(* Logix 5000 AddOnInstructionDefinition export HI1734_Faceplate_Standard_AOI; software revision 30.00 *)

ADD_ON_INSTRUCTION HI1734_Faceplate_Standard_AOI   (* revision 1.3, vendor Hardy Process solutions *)
// for standard data from module
VAR_IN_OUT
   Inp_hi1734 : HI:1734_WS:I:0; {required}   // Module Input table
   Out_hi1734 : HI:1734_WS:O:0; {required}   // Module Output table
END_VAR
VAR_OUTPUT
   cal_status : SINT; {access Read Only}   // Calibration status indication
   hardy_1734_ints_st : INT;   // Instrument Status
END_VAR
VAR_INPUT
   fp_dis_md : INT;   // display mode gross/net
   tare_cmd : BOOL;   // Tare cmd trigger
   zero_cmd : BOOL;   // Zero cmd trigger
END_VAR
VAR_OUTPUT
   hardy_1734_net_wt : REAL;   // Net weight
   hardy_1734_gross_wt : REAL;   // Gross weight
END_VAR
VAR_INPUT
   rd_fill : BOOL;   // Read Filter parameter trigger
   pm_2081 : DINT;   // WAVERSAVER
   rd_az : BOOL;   // Read zero parameters trigger
   pm_6301 : DINT;   // Auto Zero Enable
   pm_6302 : REAL;   // Auto Zero tolerance
   pm_6201 : REAL;   // zero'd weight
   pm_2886 : REAL;   // Zero Tolerance
   pm_6183 : REAL;   // Tare Weight
   rd_inst : BOOL;   // Read Instrument setup parameter trigger
   pm_2881 : DINT;   // Units of measure
   pm_2887 : REAL;   // Motion Tolerance
   rd_c2cal : BOOL;   // Read C2 parameter trigger
   pm_4102 : REAL;   // Gravity correction
   rd_tradcal : BOOL;   // Read Traditional cal parameter trigger
   pm_4182 : REAL;   // Span Weight
   cal_low_cmd : BOOL;   // Cal Low cmd trigger
   cal_high_cmd : BOOL;   // Cal High cmd trigger
   c2_cmd : BOOL;   // C2 cal trigger
END_VAR
VAR_OUTPUT
   status1 : INT;   // Instrument status
END_VAR
VAR_INPUT
   save_c2_pm : BOOL;   // Save C2 setup parameters trigger
   pm_4101 : REAL;   // Ref Weight
   save_tradcal_pm : BOOL;   // Save traditional calibration settings trigger
   save_fil_pm : BOOL;   // Save Filter settings trigger
   save_az_pm : BOOL;   // Save zero parameters trigger
   save_ins_pm : BOOL;   // Save Instrument setup settings trigger
   Set_FaceplateAnimation : INT;   // panel selection on faceplate
   pm_2082 : DINT;   // Num Averages
END_VAR
VAR_OUTPUT
   cmd_status : DINT; {access Read Only}   // Command status indication
END_VAR
VAR_INPUT
   reset_waversaver_indicator : BOOL;   // Reset WAVERSAVER selection indication on faceplate
   reset_az_enable_indication : BOOL;   // Reset auto zero selection indication on faceplate
   reset_units_indication : BOOL;   // Reset units selection indication on faceplate
   percent_weight : REAL;   // percentage of scale capacity for trend screen
   pm_2888 : REAL;   // scale capacity used for trend
END_VAR
VAR
   start_delay_rd_filter : BOOL; {access None}   // processs control bit
   delay_rd_filter : TIMER := (PRE := 200); {access None}   // Delay timer to allow time for process to complete
   rd_inst2 : BOOL; {access None}   // processs control bit
   wr_C2_ref_wt_1 : BOOL; {access None}   // processs control bit
   wr_gravity_correction_1 : BOOL; {access None}   // processs control bit
   wr_span_wt_1 : BOOL; {access None}   // processs control bit
   wr_waversaver_1 : BOOL; {access None}   // processs control bit
   wr_number_avgerages_1 : BOOL; {access None}   // processs control bit
   wr_zero_tolerance_1 : BOOL; {access None}   // processs control bit
   wr_tare_weight_1 : BOOL; {access None}   // processs control bit
   wr_motion_tolerance_1 : BOOL; {access None}   // processs control bit
   wr_units_measure_1 : BOOL; {access None}   // processs control bit
   start_delay_rd_zero_1 : BOOL; {access None}   // processs control bit
   delay_rd_zero_1 : TIMER := (PRE := 200); {access None}   // Delay timer to allow time for process to complete
   start_delay_rd_zero_2 : BOOL; {access None}   // processs control bit
   delay_rd_zero_2 : TIMER := (PRE := 200); {access None}   // Delay timer to allow time for process to complete
   start_delay_rd_inst_1 : BOOL; {access None}   // processs control bit
   delay_rd_inst_1 : TIMER := (PRE := 200); {access None}   // Delay timer to allow time for process to complete
   wr_auto_zero_enable_1 : BOOL; {access None}   // processs control bit
   wr_auto_zero_tolerance_1 : BOOL; {access None}   // processs control bit
   start_delay_rd_inst_2 : BOOL; {access None}   // processs control bit
   delay_rd_inst_2 : TIMER := (PRE := 200); {access None}   // Delay timer to allow time for process to complete
   start_delay_rd_C2cal : BOOL; {access None}   // processs control bit
   delay_rd_C2cal : TIMER := (PRE := 200); {access None}   // Delay timer to allow time for process to complete
   start_delay_rd_tradcal : BOOL; {access None}   // processs control bit
   delay_rd_tradcal : TIMER := (PRE := 200); {access None}   // Delay timer to allow time for process to complete
   cmd_no : INT; {access None}   // Cmd number being sent to module
   run_cmd : BOOL; {access None}   // processs control bit
   chec_status_wr_C2_ref : BOOL; {access None}   // triggers status check of write C2 ref
   start_delay_wr_C2_ref : BOOL; {access None}   // processs control bit
   delay_wr_C2_ref : TIMER := (PRE := 200); {access None}   // Delay timer to allow time for process to complete
   check_status_wr_gravity_correction : BOOL; {access None}   // triggers status check of write of parameter
   start_delay_wr_gravity_correction : BOOL; {access None}   // processs control bit
   delay_wr_gravity_correction : TIMER := (PRE := 200); {access None}   // Delay timer to allow time for process to complete
   wr_traditional_ref_wt_1 : BOOL; {access None}   // processs control bit
   check_status_wr_traditional_ref : BOOL; {access None}   // triggers status check of write of parameter
   start_delay_wr_traditional_ref : BOOL; {access None}   // processs control bit
   delay_wr_traditional_ref : TIMER := (PRE := 200); {access None}   // Delay timer to allow time for process to complete
   check_status_wr_span_wt : BOOL; {access None}   // triggers status check of write of parameter
   start_delay_wr_span_wt : BOOL; {access None}   // processs control bit
   delay_wr_span_wt : TIMER := (PRE := 200); {access None}   // Delay timer to allow time for process to complete
   check_status_wr_waversaver : BOOL; {access None}   // triggers status check of write of parameter
   start_delay_wr_waversaver : BOOL; {access None}   // processs control bit
   delay_wr_waversaver : TIMER := (PRE := 200); {access None}   // Delay timer to allow time for process to complete
   check_status_wr_averages : BOOL; {access None}   // triggers status check of write of parameter
   start_delay_wr_averages : BOOL; {access None}   // processs control bit
   delay_wr_averages : TIMER := (PRE := 200); {access None}   // Delay timer to allow time for process to complete
   initial_unit_rd : BOOL; {access None}   // initial read to set up initial display of units.
   check_status_wr_zero_tolerance : BOOL; {access None}   // triggers status check of write of parameter
   start_delay_wr_zero_tolerance : BOOL; {access None}   // processs control bit
   delay_wr_zero_tolerance : TIMER := (PRE := 200); {access None}   // Delay timer to allow time for process to complete
   check_status_wr_tare_weight : BOOL; {access None}   // triggers status check of write of parameter
   start_delay_wr_tare_weight : BOOL; {access None}   // processs control bit
   delay_wr_tare_weight : TIMER := (PRE := 200); {access None}   // Delay timer to allow time for process to complete
   check_status_wr_auto_zero_enable : BOOL; {access None}   // triggers status check of write parameter
   start_delay_wr_auto_zero_enable : BOOL; {access None}   // processs control bit
   delay_wr_auto_zero_enable : TIMER := (PRE := 200); {access None}   // Delay timer to allow time for process to complete
   start_delay_wr_auto_zero_tolerance : BOOL; {access None}   // processs control bit
   check_status_wr_auto_zero_tolerance : BOOL; {access None}   // triggers status check of write of parameter
   delay_wr_auto_zero_tolerance : TIMER := (PRE := 200); {access None}   // Delay timer to allow time for process to complete
   check_status_wr_motion_tolerance : BOOL; {access None}   // triggers status check of write of parameter
   start_delay_wr_motion_toleranc : BOOL; {access None}   // processs control bit
   delay_wr_motion_toleranc : TIMER := (PRE := 200); {access None}   // Delay timer to allow time for process to complete
   check_status_wr_units_measure : BOOL; {access None}   // triggers status check of write of parameter
   start_delay_wr_units_measure : BOOL; {access None}   // processs control bit
   delay_wr_units_measure : TIMER := (PRE := 200); {access None}   // Delay timer to allow time for process to complete
   start_delay_init_units_rd : BOOL; {access None}   // processs control bit
   delay_init_units_rd : TIMER := (PRE := 200); {access None}   // Delay timer to allow time for process to complete
   run_cmd_delay : TIMER := (PRE := 1000); {access None}   // Delay timer to allow time for process to complete
   rd_zero_2 : BOOL; {access None}   // processs control bit
   wr_C2_ref_wt_2 : BOOL; {access None}   // processs control bit
   wr_gravity_correction_2 : BOOL; {access None}   // processs control bit
   wr_traditional_ref_wt_2 : BOOL; {access None}   // processs control bit
   wr_span_wt_2 : BOOL; {access None}   // processs control bit
   wr_waversaver_2 : BOOL; {access None}   // processs control bit
   wr_number_avgerages_2 : BOOL; {access None}   // processs control bit
   wr_auto_zero_enable_2 : BOOL; {access None}   // processs control bit
   wr_auto_zero_tolerance_2 : BOOL; {access None}   // processs control bit
   wr_zero_tolerance_2 : BOOL; {access None}   // processs control bit
   wr_units_measure_2 : BOOL; {access None}   // processs control bit
   wr_motion_tolerance_2 : BOOL; {access None}   // processs control bit
   wr_tare_weight_2 : BOOL; {access None}   // processs control bit
   ons_1 : BOOL; {access None}   // processs control bit
   ons_2 : BOOL; {access None}   // processs control bit
   ons_3 : BOOL; {access None}   // processs control bit
   ons_4 : BOOL; {access None}   // processs control bit
   ons_5 : BOOL; {access None}   // processs control bit
   ons_6 : BOOL; {access None}   // processs control bit
   ons_7 : BOOL; {access None}   // processs control bit
   ons_8 : BOOL; {access None}   // processs control bit
   ons_9 : BOOL; {access None}   // processs control bit
   ons_10 : BOOL; {access None}   // processs control bit
   ons_11 : BOOL; {access None}   // processs control bit
   ons_12 : BOOL; {access None}   // processs control bit
   ons_13 : BOOL; {access None}   // processs control bit
   ons_14 : BOOL; {access None}   // processs control bit
   ons_15 : BOOL; {access None}   // processs control bit
   delay_reset_waversaer_ind : TIMER := (PRE := 200); {access None}   // Delay timer to allow time for process to complete
   delay_reset_az_enable_indication : TIMER := (PRE := 200); {access None}   // Delay timer to allow time for process to complete
   delay_reset_units_indication : TIMER := (PRE := 200); {access None}   // Delay timer to allow time for process to complete
END_VAR

ROUTINE Logic   (* ladder *)
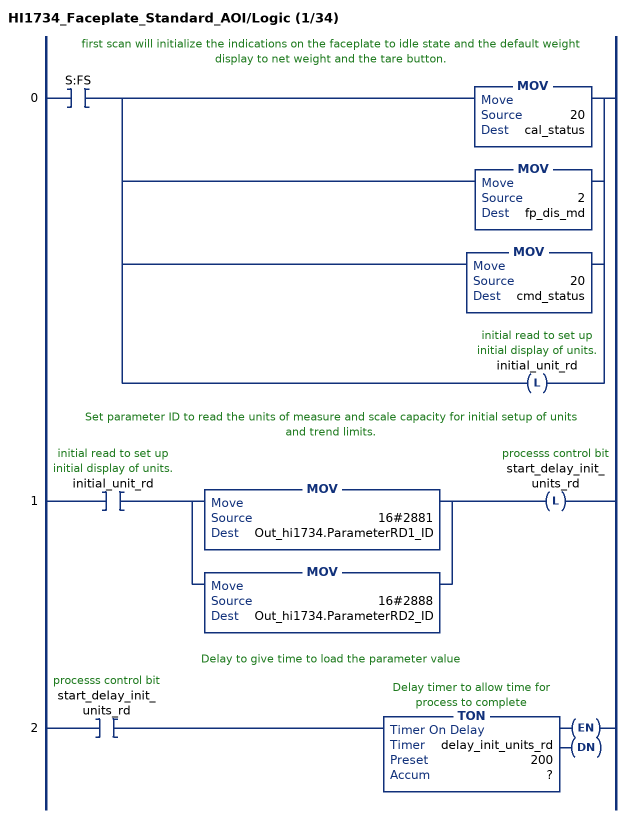
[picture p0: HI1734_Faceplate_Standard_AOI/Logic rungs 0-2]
   // first scan will initialize the indications on the faceplate to idle state and the default weight display to net weight and the tare button.
   0: XIC(S:FS)[MOV(20,cal_status) ,[MOV(2,fp_dis_md) ,MOV(20,cmd_status) ,OTL(initial_unit_rd) ] ];
   // Set parameter ID to read the units of measure and scale capacity for initial setup of units and trend limits.
   1: XIC(initial_unit_rd)[MOV(16#2881,Out_hi1734.ParameterRD1_ID) ,MOV(16#2888,Out_hi1734.ParameterRD2_ID) ]OTL(start_delay_init_units_rd);
   // Delay to give time to load the parameter value
   2: XIC(start_delay_init_units_rd)TON(delay_init_units_rd,?,?);
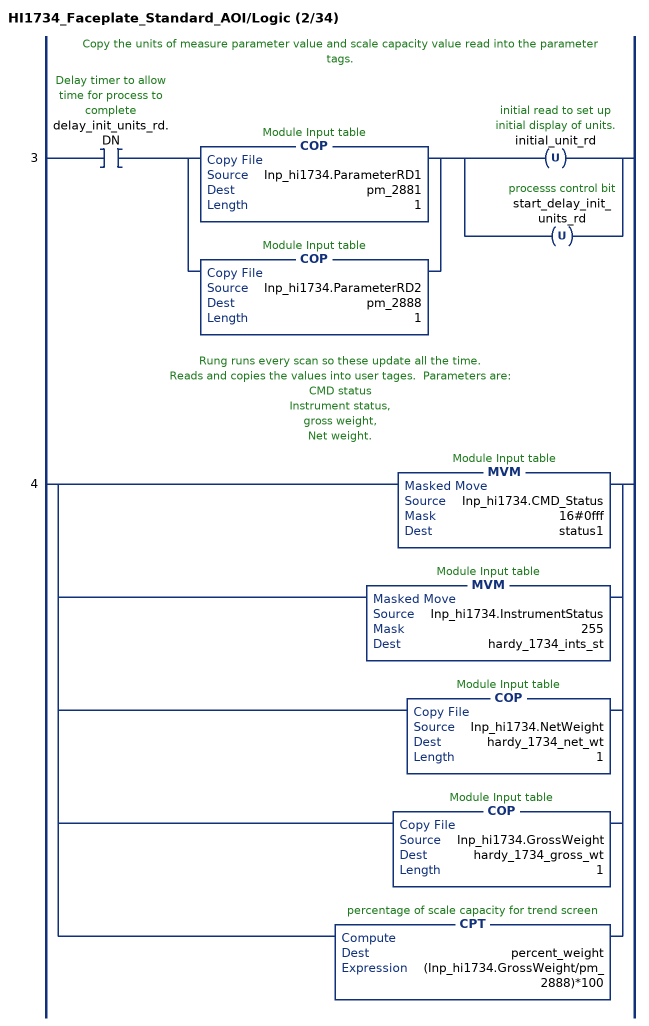
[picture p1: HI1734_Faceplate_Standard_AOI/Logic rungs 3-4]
   // Copy the units of measure parameter value and scale capacity value read into the parameter tags.
   3: XIC(delay_init_units_rd.DN)[COP(Inp_hi1734.ParameterRD1,pm_2881,1) ,COP(Inp_hi1734.ParameterRD2,pm_2888,1) ][OTU(initial_unit_rd) ,OTU(start_delay_init_units_rd) ];
   // Rung runs every scan so these update all the time.
   // Reads and copies the values into user tages.  Parameters are:
   // CMD status
   // Instrument status,
   // gross weight,
   // Net weight.
   4: [MVM(Inp_hi1734.CMD_Status,16#0fff,status1) ,MVM(Inp_hi1734.InstrumentStatus,255,hardy_1734_ints_st) ,COP(Inp_hi1734.NetWeight,hardy_1734_net_wt,1) ,COP(Inp_hi1734.GrossWeight,hardy_1734_gross_wt,1) ,CPT(percent_weight,(Inp_hi1734.GrossWeight/pm_2888)*100) ];
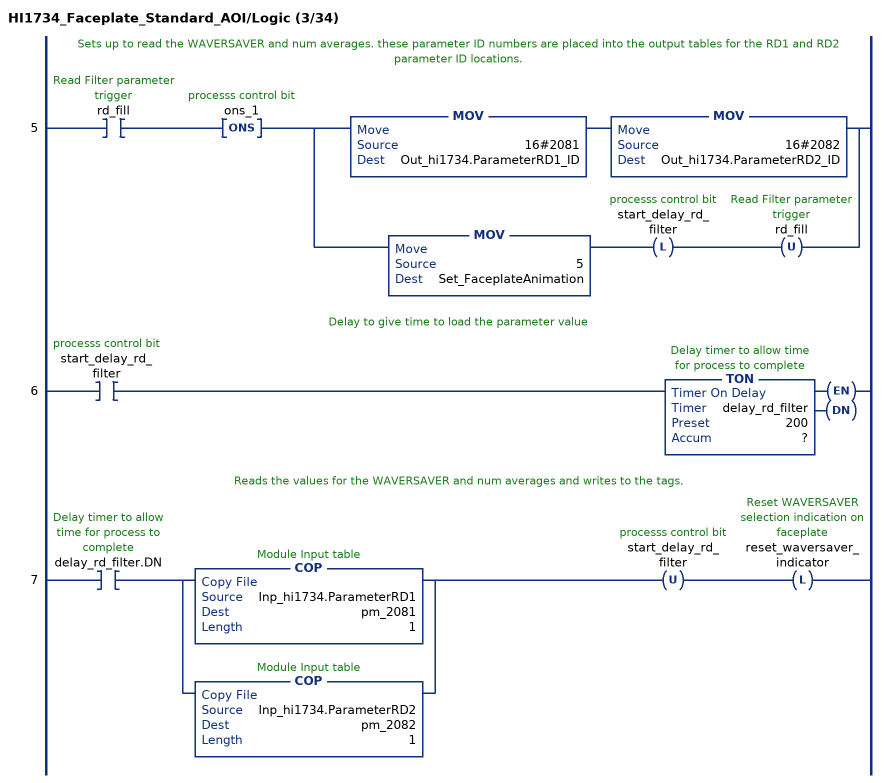
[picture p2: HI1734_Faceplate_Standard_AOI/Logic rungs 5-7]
   // Sets up to read the WAVERSAVER and num averages. these parameter ID numbers are placed into the output tables for the RD1 and RD2 parameter ID locations.
   5: XIC(rd_fill)ONS(ons_1)[MOV(16#2081,Out_hi1734.ParameterRD1_ID) MOV(16#2082,Out_hi1734.ParameterRD2_ID) ,MOV(5,Set_FaceplateAnimation) OTL(start_delay_rd_filter) OTU(rd_fill) ];
   // Delay to give time to load the parameter value
   6: XIC(start_delay_rd_filter)TON(delay_rd_filter,?,?);
   // Reads the values for the WAVERSAVER and num averages and writes to the tags.
   7: XIC(delay_rd_filter.DN)[COP(Inp_hi1734.ParameterRD1,pm_2081,1) ,COP(Inp_hi1734.ParameterRD2,pm_2082,1) ]OTU(start_delay_rd_filter)OTL(reset_waversaver_indicator);
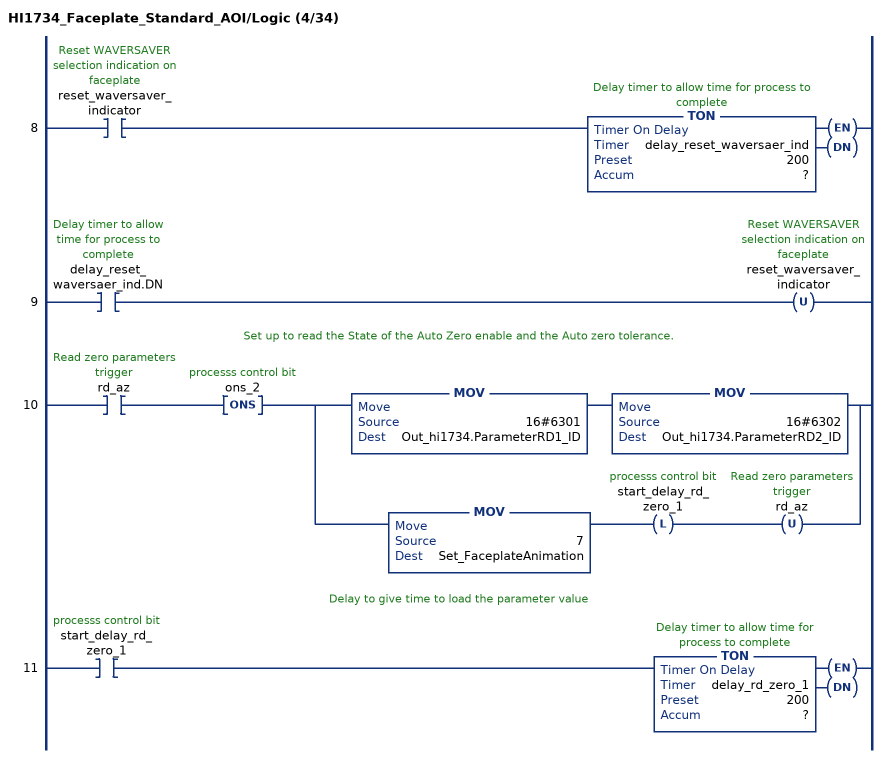
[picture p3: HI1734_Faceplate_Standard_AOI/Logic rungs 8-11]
   8: XIC(reset_waversaver_indicator)TON(delay_reset_waversaer_ind,?,?);
   9: XIC(delay_reset_waversaer_ind.DN)OTU(reset_waversaver_indicator);
   // Set up to read the State of the Auto Zero enable and the Auto zero tolerance.
   10: XIC(rd_az)ONS(ons_2)[MOV(16#6301,Out_hi1734.ParameterRD1_ID) MOV(16#6302,Out_hi1734.ParameterRD2_ID) ,MOV(7,Set_FaceplateAnimation) OTL(start_delay_rd_zero_1) OTU(rd_az) ];
   // Delay to give time to load the parameter value
   11: XIC(start_delay_rd_zero_1)TON(delay_rd_zero_1,?,?);
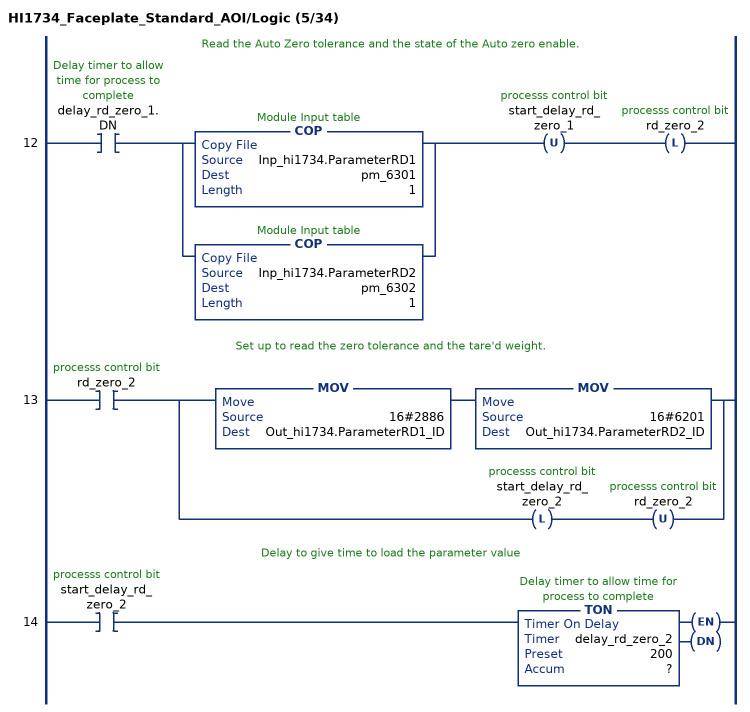
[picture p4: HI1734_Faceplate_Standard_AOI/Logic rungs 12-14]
   // Read the Auto Zero tolerance and the state of the Auto zero enable.
   12: XIC(delay_rd_zero_1.DN)[COP(Inp_hi1734.ParameterRD1,pm_6301,1) ,COP(Inp_hi1734.ParameterRD2,pm_6302,1) ]OTU(start_delay_rd_zero_1)OTL(rd_zero_2);
   // Set up to read the zero tolerance and the tare'd weight.
   13: XIC(rd_zero_2)[MOV(16#2886,Out_hi1734.ParameterRD1_ID) MOV(16#6201,Out_hi1734.ParameterRD2_ID) ,OTL(start_delay_rd_zero_2) OTU(rd_zero_2) ];
   // Delay to give time to load the parameter value
   14: XIC(start_delay_rd_zero_2)TON(delay_rd_zero_2,?,?);
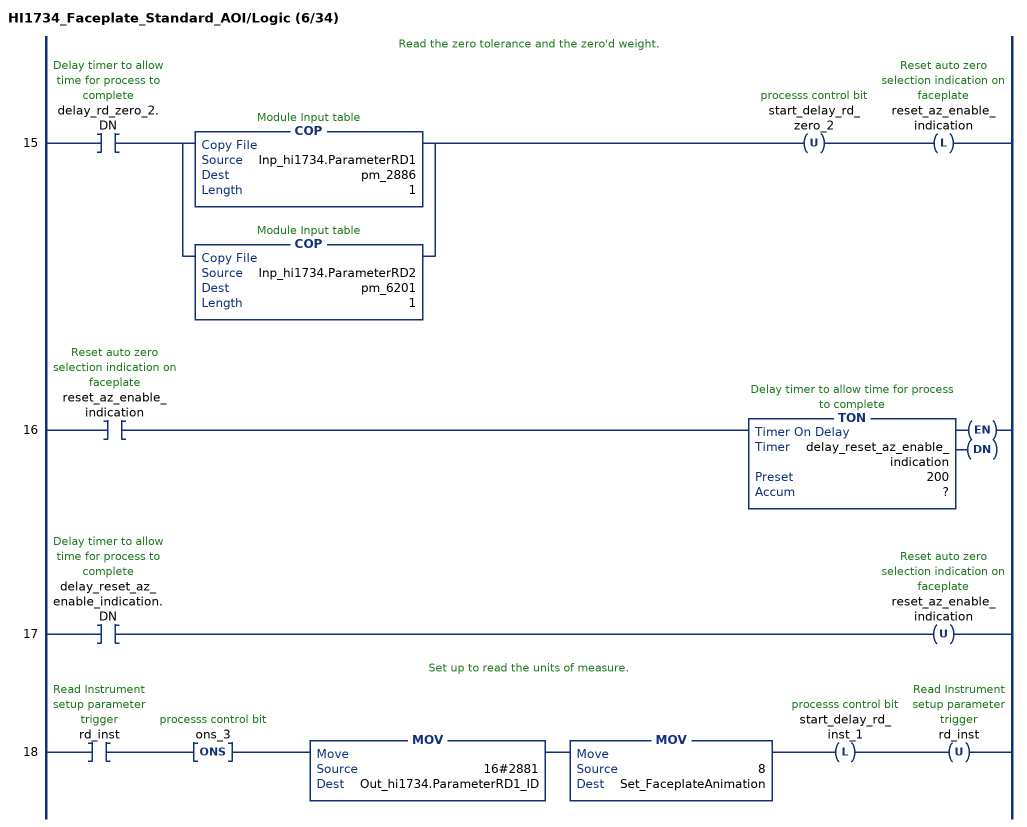
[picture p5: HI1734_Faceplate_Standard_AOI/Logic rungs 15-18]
   // Read the zero tolerance and the zero'd weight.
   15: XIC(delay_rd_zero_2.DN)[COP(Inp_hi1734.ParameterRD1,pm_2886,1) ,COP(Inp_hi1734.ParameterRD2,pm_6201,1) ]OTU(start_delay_rd_zero_2)OTL(reset_az_enable_indication);
   16: XIC(reset_az_enable_indication)TON(delay_reset_az_enable_indication,?,?);
   17: XIC(delay_reset_az_enable_indication.DN)OTU(reset_az_enable_indication);
   // Set up to read the units of measure.
   18: XIC(rd_inst)ONS(ons_3)MOV(16#2881,Out_hi1734.ParameterRD1_ID)MOV(8,Set_FaceplateAnimation)OTL(start_delay_rd_inst_1)OTU(rd_inst);
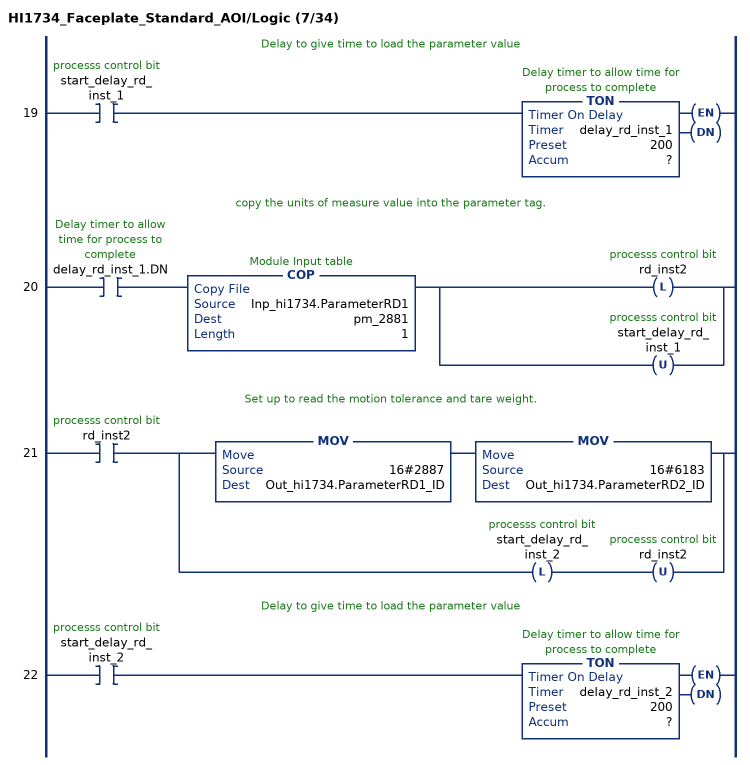
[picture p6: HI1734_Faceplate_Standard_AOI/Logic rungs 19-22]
   // Delay to give time to load the parameter value
   19: XIC(start_delay_rd_inst_1)TON(delay_rd_inst_1,?,?);
   // copy the units of measure value into the parameter tag.
   20: XIC(delay_rd_inst_1.DN)COP(Inp_hi1734.ParameterRD1,pm_2881,1)[OTL(rd_inst2) ,OTU(start_delay_rd_inst_1) ];
   // Set up to read the motion tolerance and tare weight.
   21: XIC(rd_inst2)[MOV(16#2887,Out_hi1734.ParameterRD1_ID) MOV(16#6183,Out_hi1734.ParameterRD2_ID) ,OTL(start_delay_rd_inst_2) OTU(rd_inst2) ];
   // Delay to give time to load the parameter value
   22: XIC(start_delay_rd_inst_2)TON(delay_rd_inst_2,?,?);
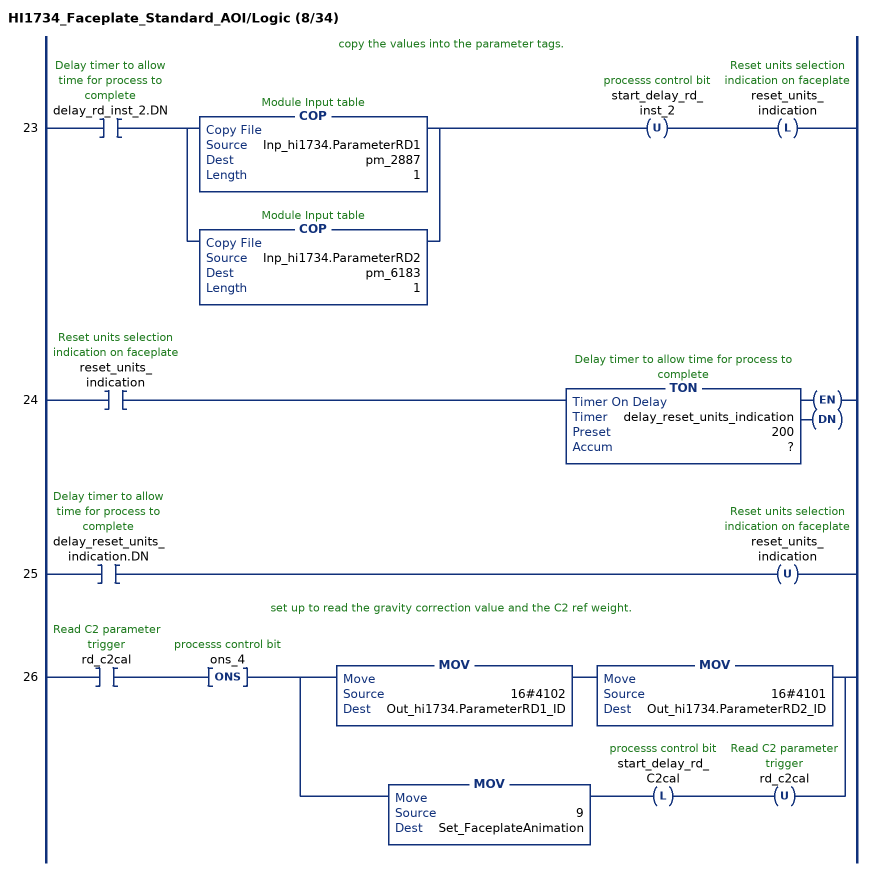
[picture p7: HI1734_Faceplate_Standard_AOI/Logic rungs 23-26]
   // copy the values into the parameter tags.
   23: XIC(delay_rd_inst_2.DN)[COP(Inp_hi1734.ParameterRD1,pm_2887,1) ,COP(Inp_hi1734.ParameterRD2,pm_6183,1) ]OTU(start_delay_rd_inst_2)OTL(reset_units_indication);
   24: XIC(reset_units_indication)TON(delay_reset_units_indication,?,?);
   25: XIC(delay_reset_units_indication.DN)OTU(reset_units_indication);
   // set up to read the gravity correction value and the C2 ref weight.
   26: XIC(rd_c2cal)ONS(ons_4)[MOV(16#4102,Out_hi1734.ParameterRD1_ID) MOV(16#4101,Out_hi1734.ParameterRD2_ID) ,MOV(9,Set_FaceplateAnimation) OTL(start_delay_rd_C2cal) OTU(rd_c2cal) ];
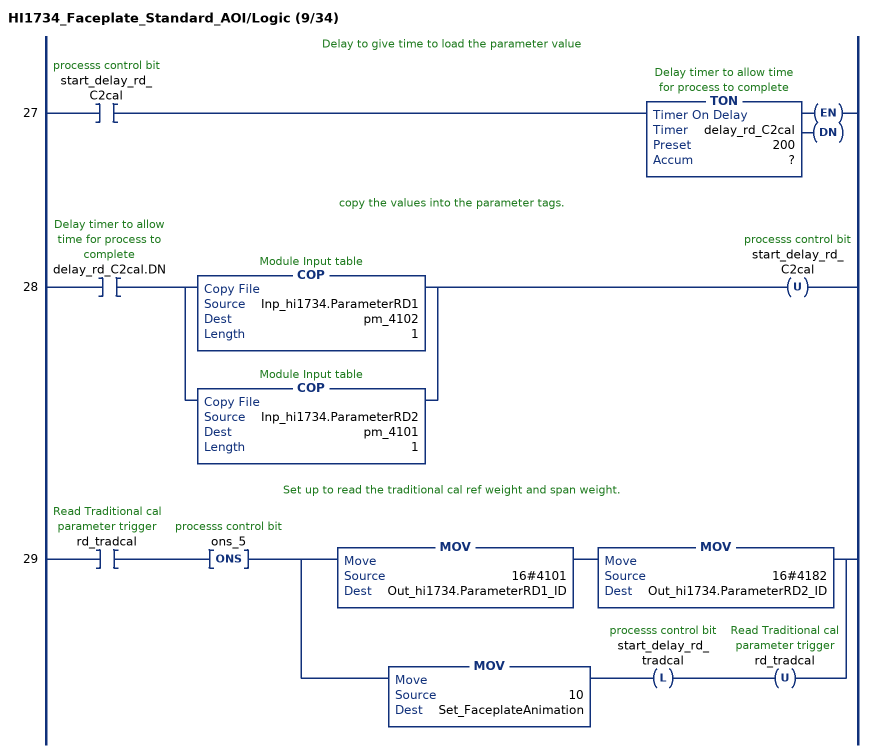
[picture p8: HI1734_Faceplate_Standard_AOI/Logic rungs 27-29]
   // Delay to give time to load the parameter value
   27: XIC(start_delay_rd_C2cal)TON(delay_rd_C2cal,?,?);
   // copy the values into the parameter tags.
   28: XIC(delay_rd_C2cal.DN)[COP(Inp_hi1734.ParameterRD1,pm_4102,1) ,COP(Inp_hi1734.ParameterRD2,pm_4101,1) ]OTU(start_delay_rd_C2cal);
   // Set up to read the traditional cal ref weight and span weight.
   29: XIC(rd_tradcal)ONS(ons_5)[MOV(16#4101,Out_hi1734.ParameterRD1_ID) MOV(16#4182,Out_hi1734.ParameterRD2_ID) ,MOV(10,Set_FaceplateAnimation) OTL(start_delay_rd_tradcal) OTU(rd_tradcal) ];
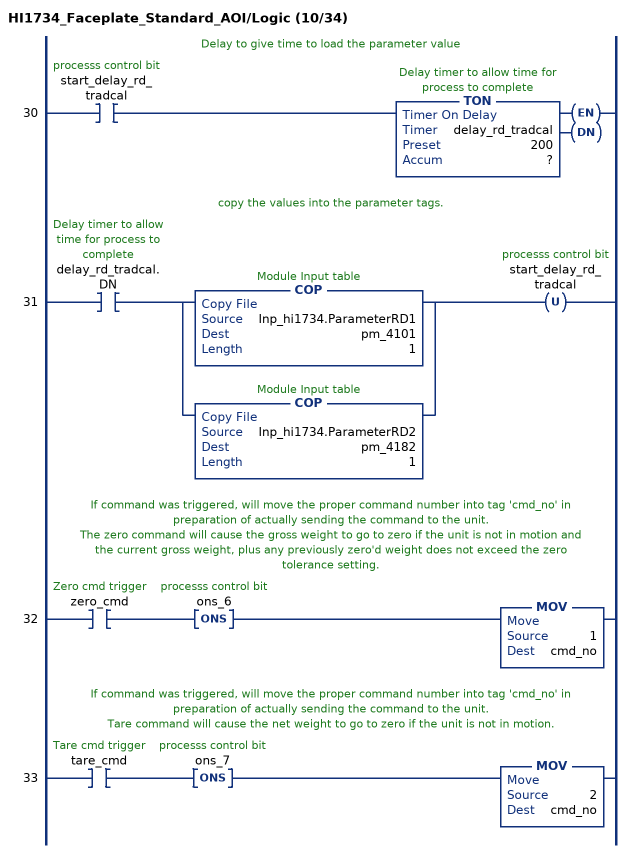
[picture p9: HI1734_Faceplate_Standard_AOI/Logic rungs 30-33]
   // Delay to give time to load the parameter value
   30: XIC(start_delay_rd_tradcal)TON(delay_rd_tradcal,?,?);
   // copy the values into the parameter tags.
   31: XIC(delay_rd_tradcal.DN)[COP(Inp_hi1734.ParameterRD1,pm_4101,1) ,COP(Inp_hi1734.ParameterRD2,pm_4182,1) ]OTU(start_delay_rd_tradcal);
   // If command was triggered, will move the proper command number into tag 'cmd_no' in preparation of actually sending the command to the unit.
   // The zero command will cause the gross weight to go to zero if the unit is not in motion and the current gross weight, plus any previously zero'd weight does not exceed the zero tolerance setting.
   32: XIC(zero_cmd)ONS(ons_6)MOV(1,cmd_no);
   // If command was triggered, will move the proper command number into tag 'cmd_no' in preparation of actually sending the command to the unit.
   // Tare command will cause the net weight to go to zero if the unit is not in motion.
   33: XIC(tare_cmd)ONS(ons_7)MOV(2,cmd_no);
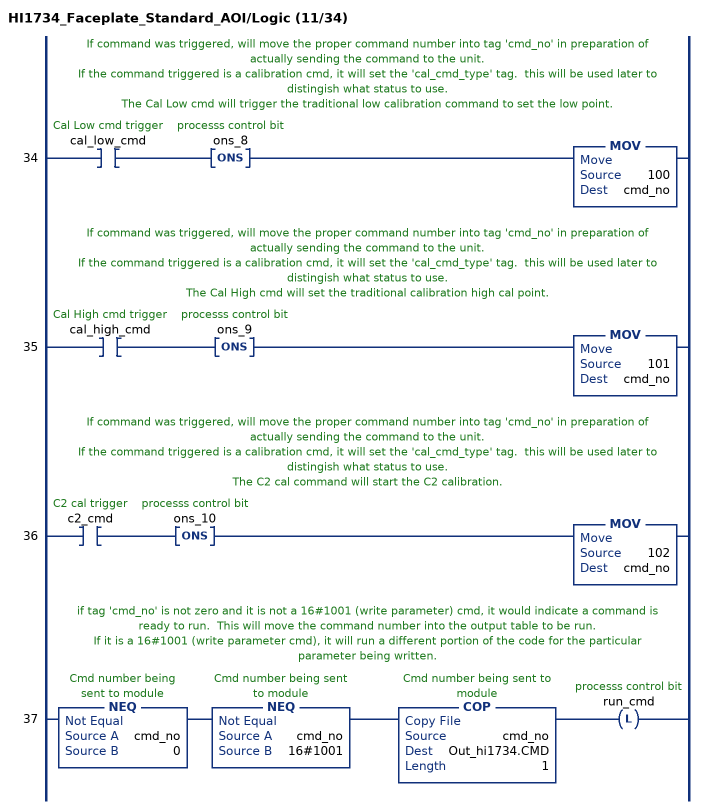
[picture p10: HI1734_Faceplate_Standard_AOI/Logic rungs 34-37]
   // If command was triggered, will move the proper command number into tag 'cmd_no' in preparation of actually sending the command to the unit.
   // If the command triggered is a calibration cmd, it will set the 'cal_cmd_type' tag.  this will be used later to distingish what status to use.
   // The Cal Low cmd will trigger the traditional low calibration command to set the low point.
   34: XIC(cal_low_cmd)ONS(ons_8)MOV(100,cmd_no);
   // If command was triggered, will move the proper command number into tag 'cmd_no' in preparation of actually sending the command to the unit.
   // If the command triggered is a calibration cmd, it will set the 'cal_cmd_type' tag.  this will be used later to distingish what status to use.
   // The Cal High cmd will set the traditional calibration high cal point.
   35: XIC(cal_high_cmd)ONS(ons_9)MOV(101,cmd_no);
   // If command was triggered, will move the proper command number into tag 'cmd_no' in preparation of actually sending the command to the unit.
   // If the command triggered is a calibration cmd, it will set the 'cal_cmd_type' tag.  this will be used later to distingish what status to use.
   // The C2 cal command will start the C2 calibration.
   36: XIC(c2_cmd)ONS(ons_10)MOV(102,cmd_no);
   // if tag 'cmd_no' is not zero and it is not a 16#1001 (write parameter) cmd, it would indicate a command is ready to run.  This will move the command number into the output table to be run.
   // If it is a 16#1001 (write parameter cmd), it will run a different portion of the code for the particular parameter being written.
   37: NEQ(cmd_no,0)NEQ(cmd_no,16#1001)COP(cmd_no,Out_hi1734.CMD,1)OTL(run_cmd);
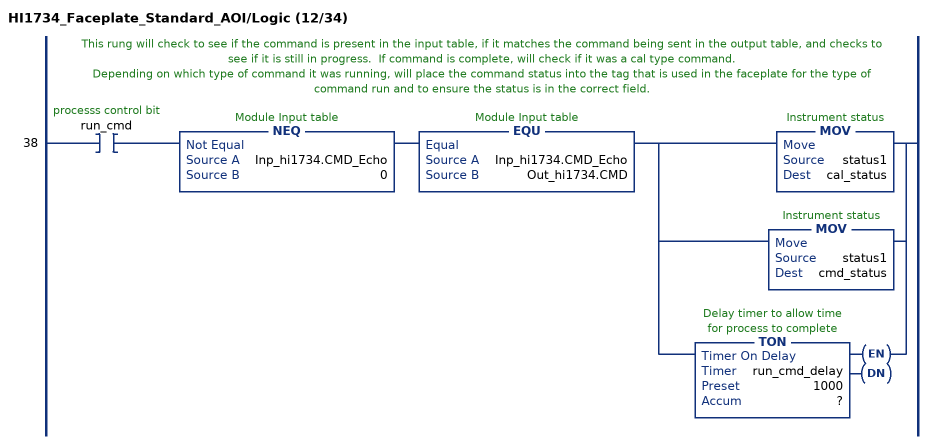
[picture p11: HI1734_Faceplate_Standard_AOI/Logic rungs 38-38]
   // This rung will check to see if the command is present in the input table, if it matches the command being sent in the output table, and checks to see if it is still in progress.  If command is complete, will check if it was a cal type command.
   // Depending on which type of command it was running, will place the command status into the tag that is used in the faceplate for the type of command run and to ensure the status is in the correct field.
   38: XIC(run_cmd)NEQ(Inp_hi1734.CMD_Echo,0)EQU(Inp_hi1734.CMD_Echo,Out_hi1734.CMD)[MOV(status1,cal_status) ,MOV(status1,cmd_status) ,TON(run_cmd_delay,?,?) ];
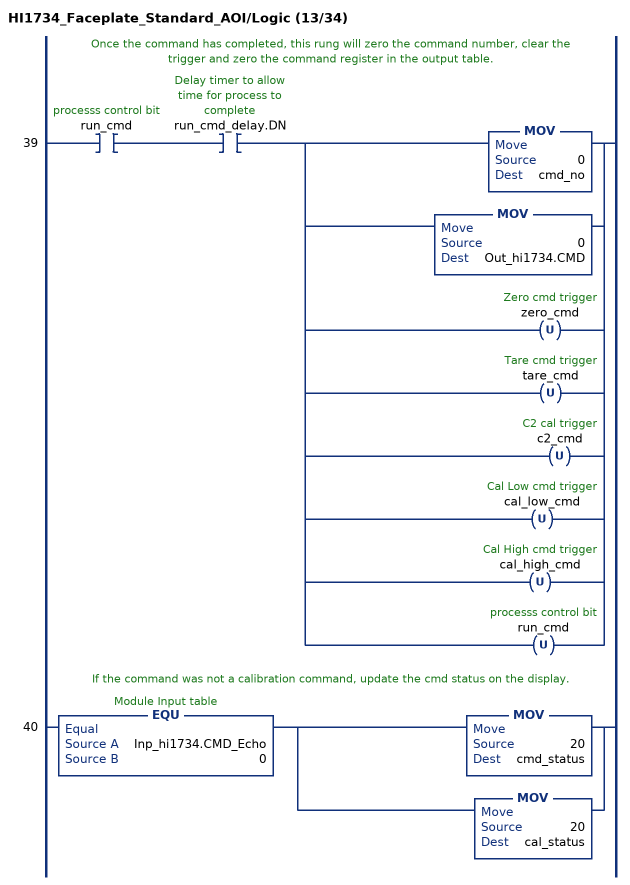
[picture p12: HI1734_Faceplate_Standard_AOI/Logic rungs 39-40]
   // Once the command has completed, this rung will zero the command number, clear the trigger and zero the command register in the output table.
   39: XIC(run_cmd)XIC(run_cmd_delay.DN)[MOV(0,cmd_no) ,MOV(0,Out_hi1734.CMD) ,OTU(zero_cmd) ,OTU(tare_cmd) ,OTU(c2_cmd) ,OTU(cal_low_cmd) ,OTU(cal_high_cmd) ,OTU(run_cmd) ];
   // If the command was not a calibration command, update the cmd status on the display.
   40: EQU(Inp_hi1734.CMD_Echo,0)[MOV(20,cmd_status) ,MOV(20,cal_status) ];
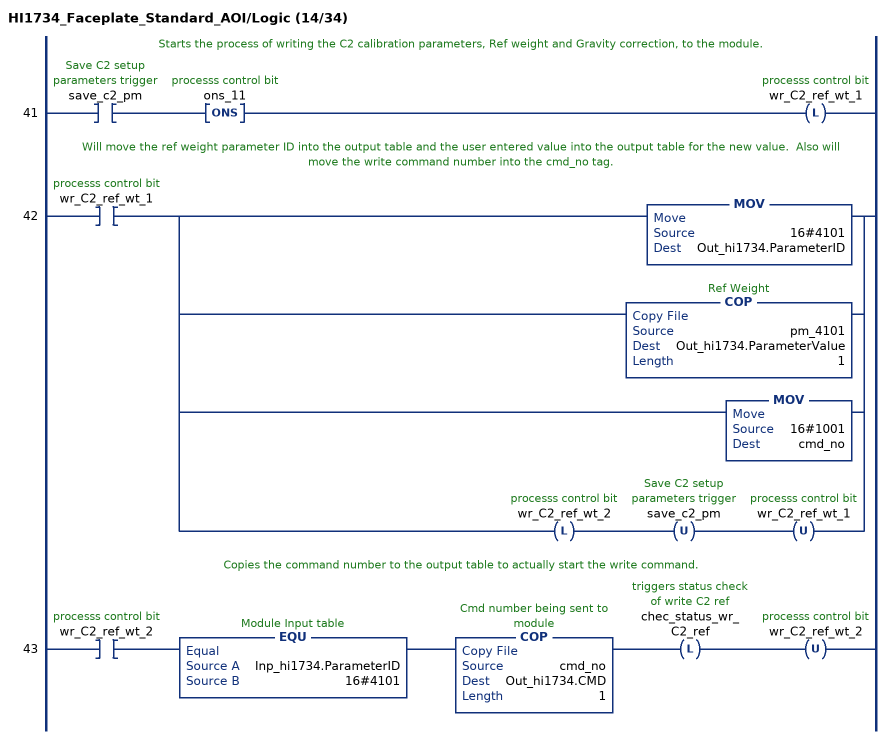
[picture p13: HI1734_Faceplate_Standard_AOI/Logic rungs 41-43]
   // Starts the process of writing the C2 calibration parameters, Ref weight and Gravity correction, to the module.
   41: XIC(save_c2_pm)ONS(ons_11)OTL(wr_C2_ref_wt_1);
   // Will move the ref weight parameter ID into the output table and the user entered value into the output table for the new value.  Also will move the write command number into the cmd_no tag.
   42: XIC(wr_C2_ref_wt_1)[MOV(16#4101,Out_hi1734.ParameterID) ,COP(pm_4101,Out_hi1734.ParameterValue,1) ,MOV(16#1001,cmd_no) ,OTL(wr_C2_ref_wt_2) OTU(save_c2_pm) OTU(wr_C2_ref_wt_1) ];
   // Copies the command number to the output table to actually start the write command.
   43: XIC(wr_C2_ref_wt_2)EQU(Inp_hi1734.ParameterID,16#4101)COP(cmd_no,Out_hi1734.CMD,1)OTL(chec_status_wr_C2_ref)OTU(wr_C2_ref_wt_2);
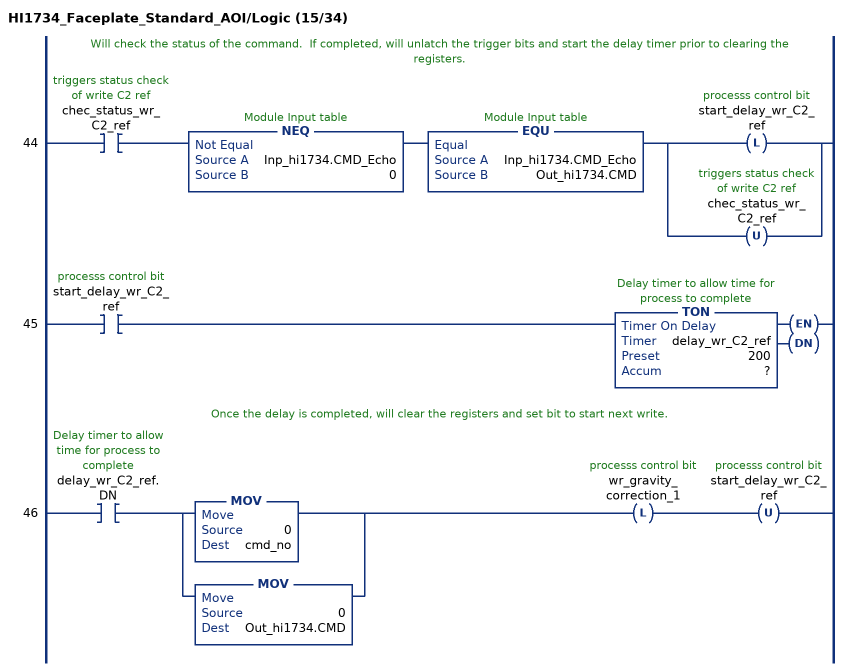
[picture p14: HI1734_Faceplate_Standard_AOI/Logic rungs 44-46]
   // Will check the status of the command.  If completed, will unlatch the trigger bits and start the delay timer prior to clearing the registers.
   44: XIC(chec_status_wr_C2_ref)NEQ(Inp_hi1734.CMD_Echo,0)EQU(Inp_hi1734.CMD_Echo,Out_hi1734.CMD)[OTL(start_delay_wr_C2_ref) ,OTU(chec_status_wr_C2_ref) ];
   45: XIC(start_delay_wr_C2_ref)TON(delay_wr_C2_ref,?,?);
   // Once the delay is completed, will clear the registers and set bit to start next write.
   46: XIC(delay_wr_C2_ref.DN)[MOV(0,cmd_no) ,MOV(0,Out_hi1734.CMD) ]OTL(wr_gravity_correction_1)OTU(start_delay_wr_C2_ref);
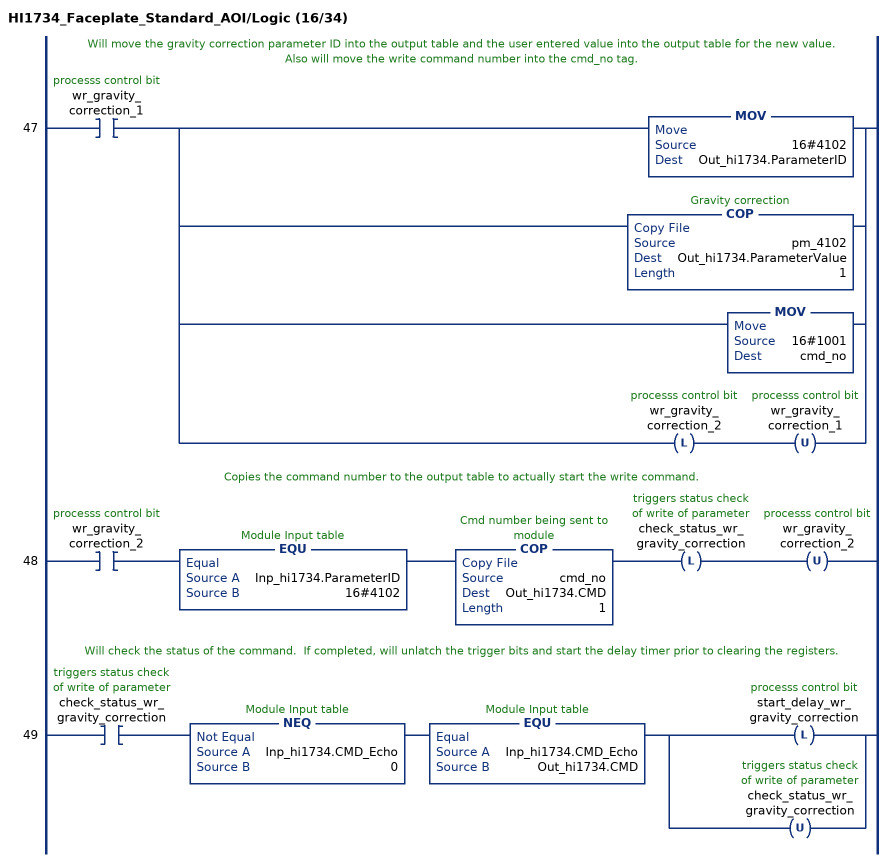
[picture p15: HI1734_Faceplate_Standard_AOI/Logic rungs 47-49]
   // Will move the gravity correction parameter ID into the output table and the user entered value into the output table for the new value.  Also will move the write command number into the cmd_no tag.
   47: XIC(wr_gravity_correction_1)[MOV(16#4102,Out_hi1734.ParameterID) ,COP(pm_4102,Out_hi1734.ParameterValue,1) ,MOV(16#1001,cmd_no) ,OTL(wr_gravity_correction_2) OTU(wr_gravity_correction_1) ];
   // Copies the command number to the output table to actually start the write command.
   48: XIC(wr_gravity_correction_2)EQU(Inp_hi1734.ParameterID,16#4102)COP(cmd_no,Out_hi1734.CMD,1)OTL(check_status_wr_gravity_correction)OTU(wr_gravity_correction_2);
   // Will check the status of the command.  If completed, will unlatch the trigger bits and start the delay timer prior to clearing the registers.
   49: XIC(check_status_wr_gravity_correction)NEQ(Inp_hi1734.CMD_Echo,0)EQU(Inp_hi1734.CMD_Echo,Out_hi1734.CMD)[OTL(start_delay_wr_gravity_correction) ,OTU(check_status_wr_gravity_correction) ];
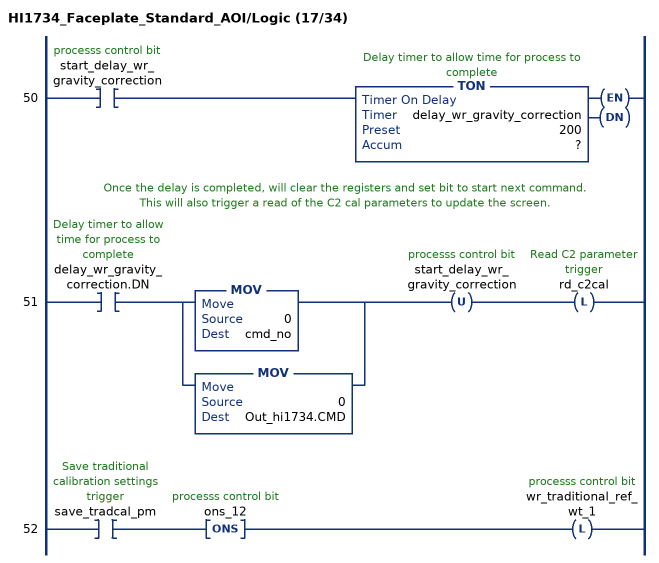
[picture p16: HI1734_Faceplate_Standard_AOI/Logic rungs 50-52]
   50: XIC(start_delay_wr_gravity_correction)TON(delay_wr_gravity_correction,?,?);
   // Once the delay is completed, will clear the registers and set bit to start next command.
   // This will also trigger a read of the C2 cal parameters to update the screen.
   51: XIC(delay_wr_gravity_correction.DN)[MOV(0,cmd_no) ,MOV(0,Out_hi1734.CMD) ]OTU(start_delay_wr_gravity_correction)OTL(rd_c2cal);
   52: XIC(save_tradcal_pm)ONS(ons_12)OTL(wr_traditional_ref_wt_1);
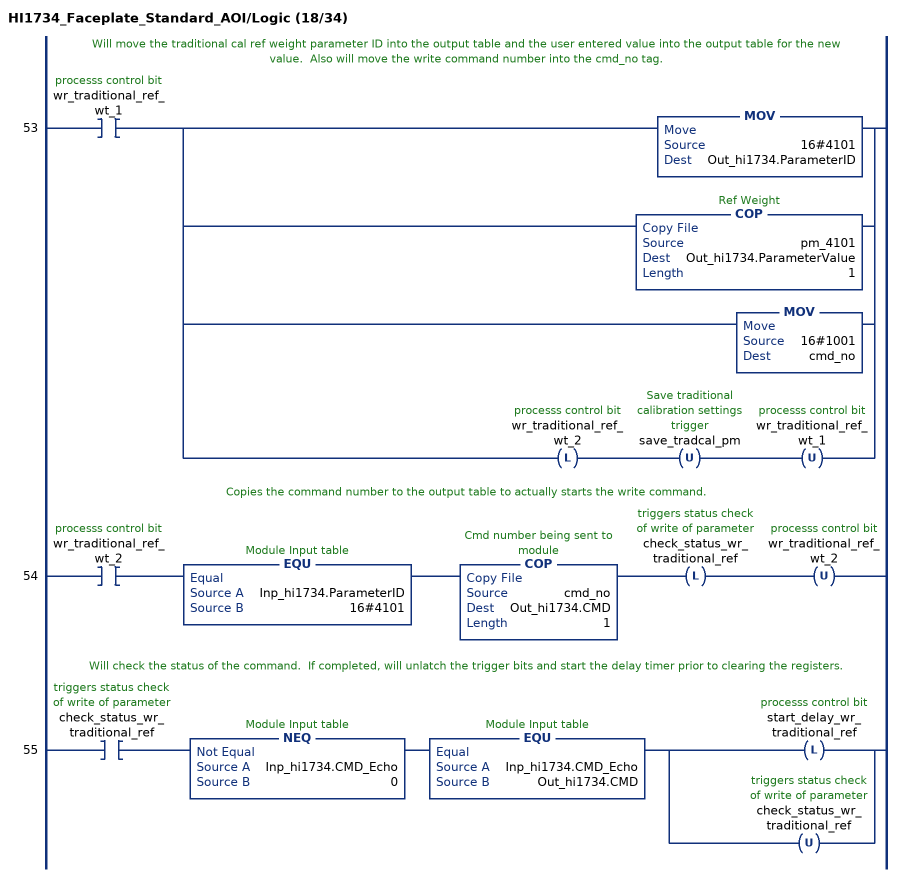
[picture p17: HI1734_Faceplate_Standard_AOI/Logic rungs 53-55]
   // Will move the traditional cal ref weight parameter ID into the output table and the user entered value into the output table for the new value.  Also will move the write command number into the cmd_no tag.
   53: XIC(wr_traditional_ref_wt_1)[MOV(16#4101,Out_hi1734.ParameterID) ,COP(pm_4101,Out_hi1734.ParameterValue,1) ,MOV(16#1001,cmd_no) ,OTL(wr_traditional_ref_wt_2) OTU(save_tradcal_pm) OTU(wr_traditional_ref_wt_1) ];
   // Copies the command number to the output table to actually starts the write command.
   54: XIC(wr_traditional_ref_wt_2)EQU(Inp_hi1734.ParameterID,16#4101)COP(cmd_no,Out_hi1734.CMD,1)OTL(check_status_wr_traditional_ref)OTU(wr_traditional_ref_wt_2);
   // Will check the status of the command.  If completed, will unlatch the trigger bits and start the delay timer prior to clearing the registers.
   55: XIC(check_status_wr_traditional_ref)NEQ(Inp_hi1734.CMD_Echo,0)EQU(Inp_hi1734.CMD_Echo,Out_hi1734.CMD)[OTL(start_delay_wr_traditional_ref) ,OTU(check_status_wr_traditional_ref) ];
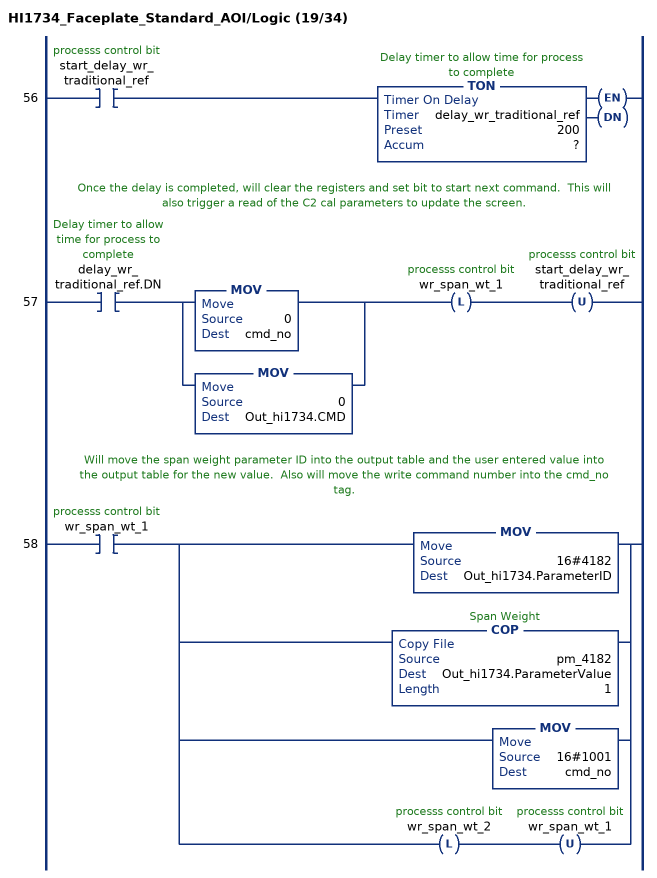
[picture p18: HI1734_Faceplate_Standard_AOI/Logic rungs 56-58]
   56: XIC(start_delay_wr_traditional_ref)TON(delay_wr_traditional_ref,?,?);
   // Once the delay is completed, will clear the registers and set bit to start next command.  This will also trigger a read of the C2 cal parameters to update the screen.
   57: XIC(delay_wr_traditional_ref.DN)[MOV(0,cmd_no) ,MOV(0,Out_hi1734.CMD) ]OTL(wr_span_wt_1)OTU(start_delay_wr_traditional_ref);
   // Will move the span weight parameter ID into the output table and the user entered value into the output table for the new value.  Also will move the write command number into the cmd_no tag.
   58: XIC(wr_span_wt_1)[MOV(16#4182,Out_hi1734.ParameterID) ,COP(pm_4182,Out_hi1734.ParameterValue,1) ,MOV(16#1001,cmd_no) ,OTL(wr_span_wt_2) OTU(wr_span_wt_1) ];
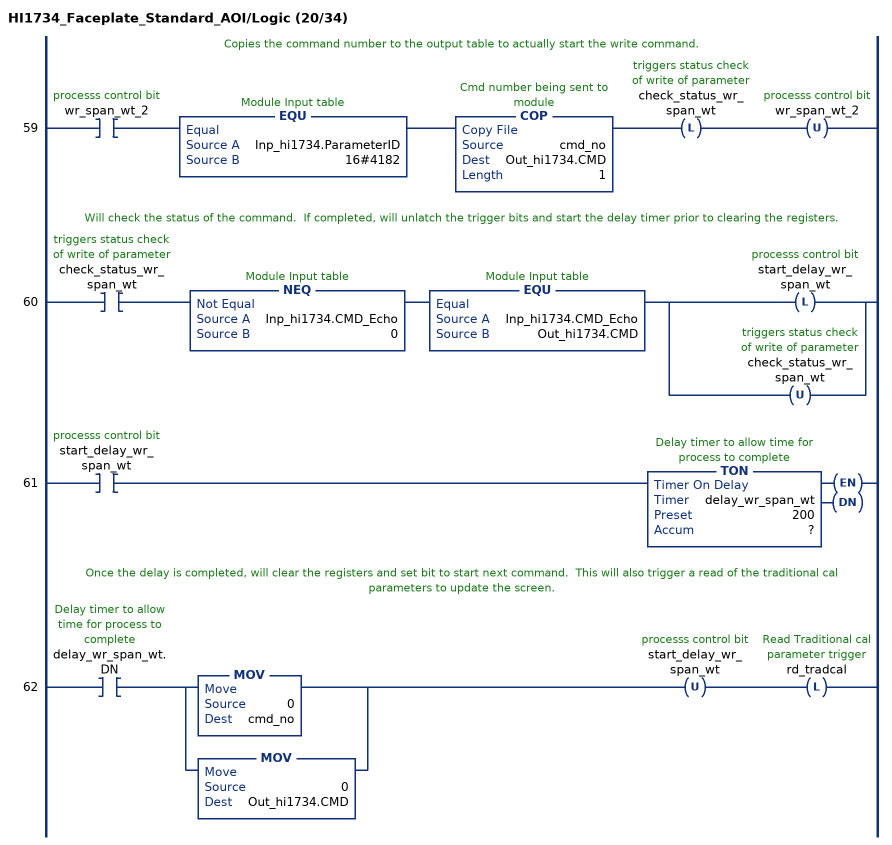
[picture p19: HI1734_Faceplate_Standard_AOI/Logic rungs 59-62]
   // Copies the command number to the output table to actually start the write command.
   59: XIC(wr_span_wt_2)EQU(Inp_hi1734.ParameterID,16#4182)COP(cmd_no,Out_hi1734.CMD,1)OTL(check_status_wr_span_wt)OTU(wr_span_wt_2);
   // Will check the status of the command.  If completed, will unlatch the trigger bits and start the delay timer prior to clearing the registers.
   60: XIC(check_status_wr_span_wt)NEQ(Inp_hi1734.CMD_Echo,0)EQU(Inp_hi1734.CMD_Echo,Out_hi1734.CMD)[OTL(start_delay_wr_span_wt) ,OTU(check_status_wr_span_wt) ];
   61: XIC(start_delay_wr_span_wt)TON(delay_wr_span_wt,?,?);
   // Once the delay is completed, will clear the registers and set bit to start next command.  This will also trigger a read of the traditional cal parameters to update the screen.
   62: XIC(delay_wr_span_wt.DN)[MOV(0,cmd_no) ,MOV(0,Out_hi1734.CMD) ]OTU(start_delay_wr_span_wt)OTL(rd_tradcal);
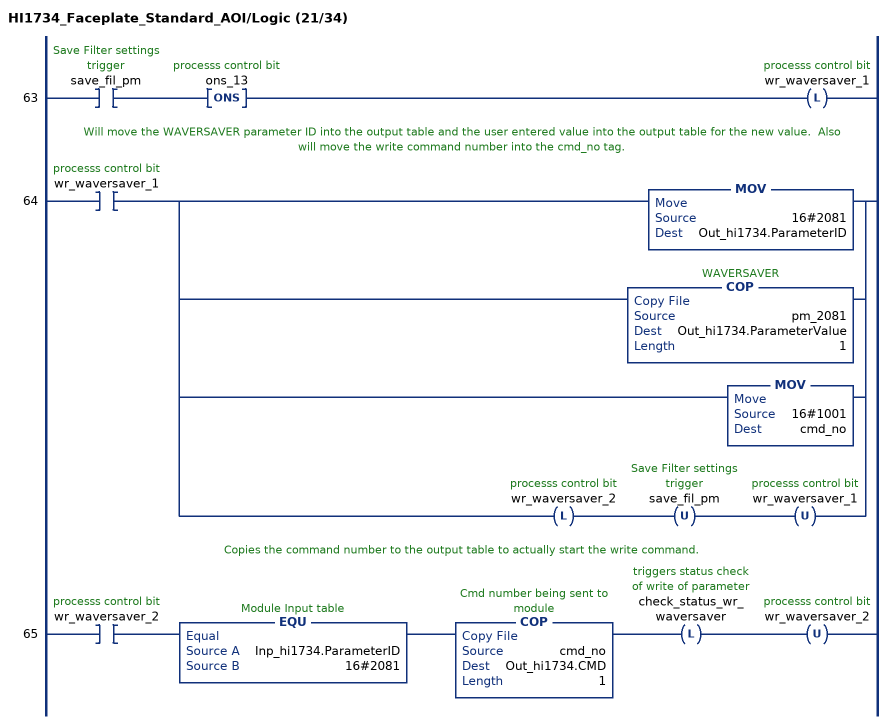
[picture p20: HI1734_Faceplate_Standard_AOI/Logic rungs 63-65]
   63: XIC(save_fil_pm)ONS(ons_13)OTL(wr_waversaver_1);
   // Will move the WAVERSAVER parameter ID into the output table and the user entered value into the output table for the new value.  Also will move the write command number into the cmd_no tag.
   64: XIC(wr_waversaver_1)[MOV(16#2081,Out_hi1734.ParameterID) ,COP(pm_2081,Out_hi1734.ParameterValue,1) ,MOV(16#1001,cmd_no) ,OTL(wr_waversaver_2) OTU(save_fil_pm) OTU(wr_waversaver_1) ];
   // Copies the command number to the output table to actually start the write command.
   65: XIC(wr_waversaver_2)EQU(Inp_hi1734.ParameterID,16#2081)COP(cmd_no,Out_hi1734.CMD,1)OTL(check_status_wr_waversaver)OTU(wr_waversaver_2);
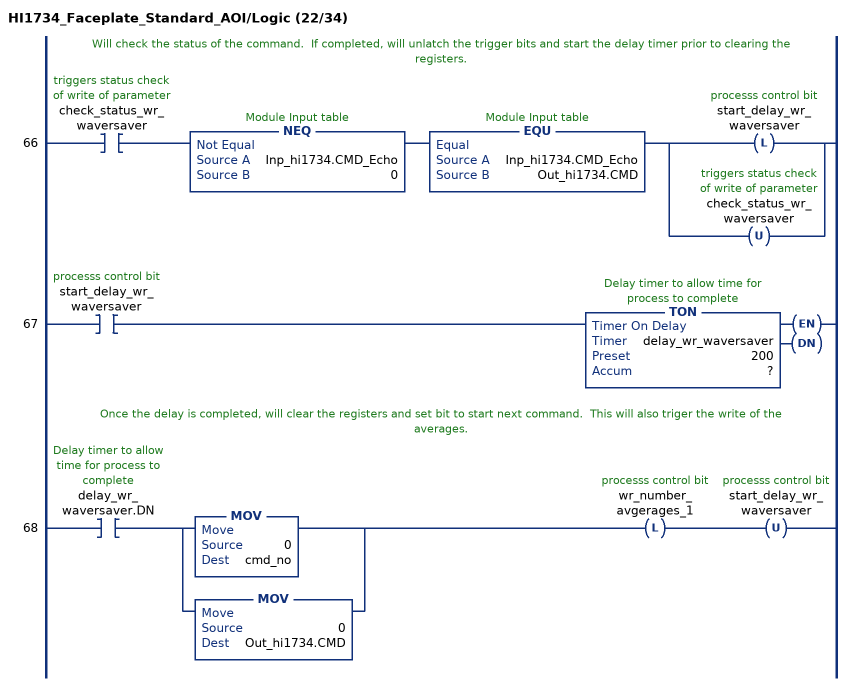
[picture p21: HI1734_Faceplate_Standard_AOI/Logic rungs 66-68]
   // Will check the status of the command.  If completed, will unlatch the trigger bits and start the delay timer prior to clearing the registers.
   66: XIC(check_status_wr_waversaver)NEQ(Inp_hi1734.CMD_Echo,0)EQU(Inp_hi1734.CMD_Echo,Out_hi1734.CMD)[OTL(start_delay_wr_waversaver) ,OTU(check_status_wr_waversaver) ];
   67: XIC(start_delay_wr_waversaver)TON(delay_wr_waversaver,?,?);
   // Once the delay is completed, will clear the registers and set bit to start next command.  This will also triger the write of the averages.
   68: XIC(delay_wr_waversaver.DN)[MOV(0,cmd_no) ,MOV(0,Out_hi1734.CMD) ]OTL(wr_number_avgerages_1)OTU(start_delay_wr_waversaver);
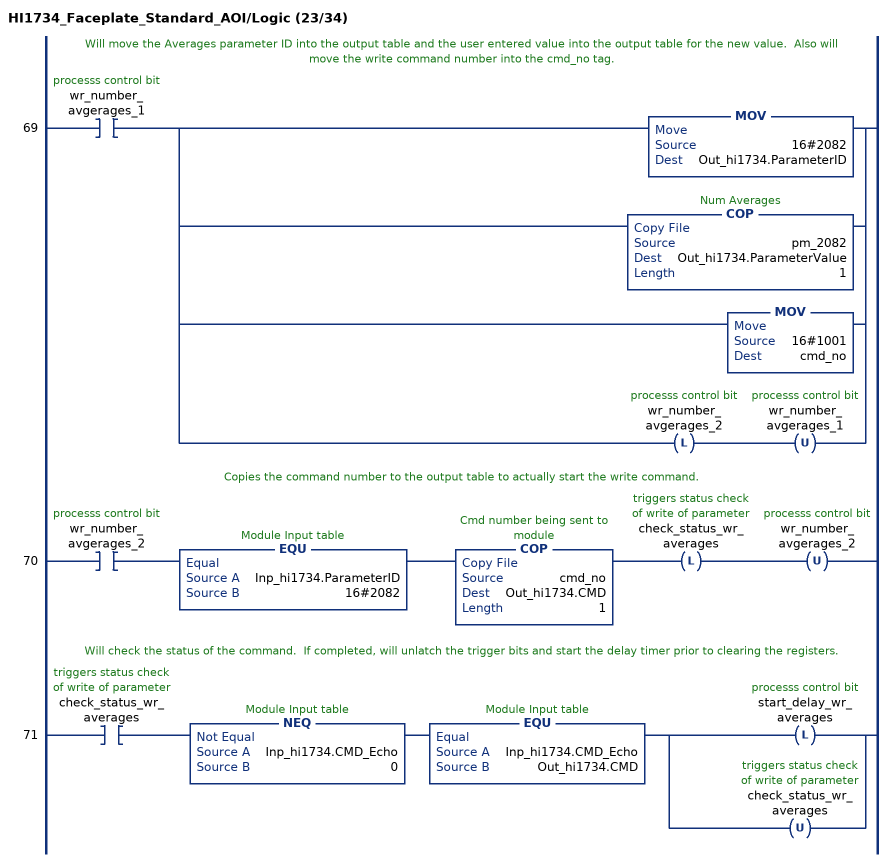
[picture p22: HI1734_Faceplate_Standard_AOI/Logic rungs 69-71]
   // Will move the Averages parameter ID into the output table and the user entered value into the output table for the new value.  Also will move the write command number into the cmd_no tag.
   69: XIC(wr_number_avgerages_1)[MOV(16#2082,Out_hi1734.ParameterID) ,COP(pm_2082,Out_hi1734.ParameterValue,1) ,MOV(16#1001,cmd_no) ,OTL(wr_number_avgerages_2) OTU(wr_number_avgerages_1) ];
   // Copies the command number to the output table to actually start the write command.
   70: XIC(wr_number_avgerages_2)EQU(Inp_hi1734.ParameterID,16#2082)COP(cmd_no,Out_hi1734.CMD,1)OTL(check_status_wr_averages)OTU(wr_number_avgerages_2);
   // Will check the status of the command.  If completed, will unlatch the trigger bits and start the delay timer prior to clearing the registers.
   71: XIC(check_status_wr_averages)NEQ(Inp_hi1734.CMD_Echo,0)EQU(Inp_hi1734.CMD_Echo,Out_hi1734.CMD)[OTL(start_delay_wr_averages) ,OTU(check_status_wr_averages) ];
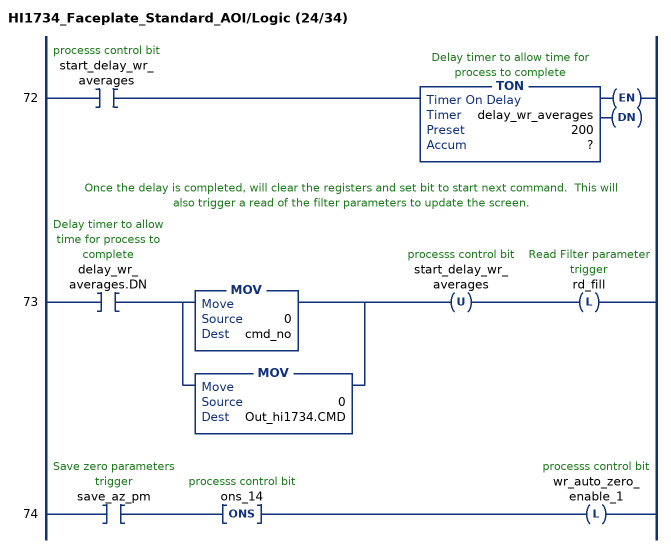
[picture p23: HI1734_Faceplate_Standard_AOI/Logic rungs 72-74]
   72: XIC(start_delay_wr_averages)TON(delay_wr_averages,?,?);
   // Once the delay is completed, will clear the registers and set bit to start next command.  This will also trigger a read of the filter parameters to update the screen.
   73: XIC(delay_wr_averages.DN)[MOV(0,cmd_no) ,MOV(0,Out_hi1734.CMD) ]OTU(start_delay_wr_averages)OTL(rd_fill);
   74: XIC(save_az_pm)ONS(ons_14)OTL(wr_auto_zero_enable_1);
